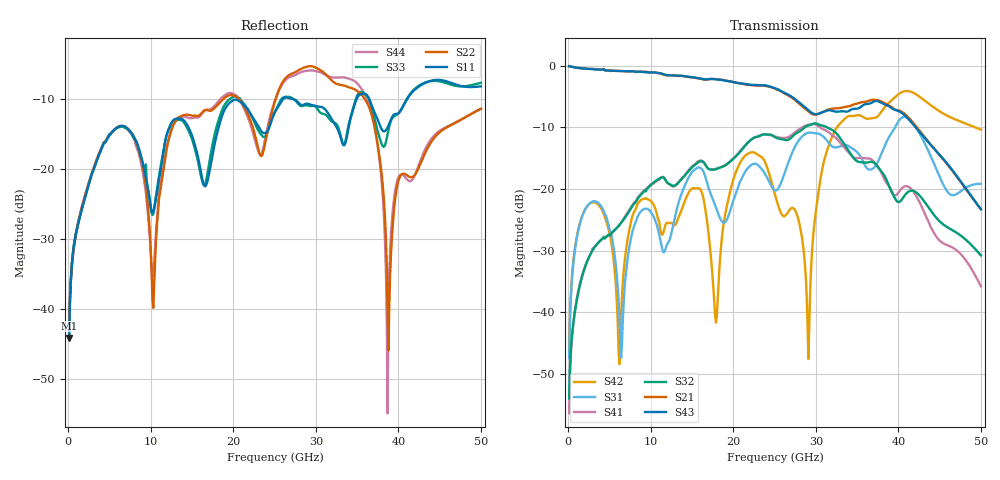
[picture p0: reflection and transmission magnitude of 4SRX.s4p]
! DAC39RF10ACK
! 256-pin FCBGA package
! Texas Instruments 8/20/2022
! Single-ended  S-parameters
! PORT#  PORT_NAME  NET_NAME
! PORT1:  xSRXN.DIEBUMP  xSRXN
! PORT2:  xSRXN.BGA  xSRXN
! PORT3:  xSRXP.DIEBUMP  xSRXP
! PORT4:  xSRXP.BGA  xSRXP
! Touchstone Ver. 1.0
! Number of ports is 4
# Hz	S	MA	R	50.000000
! SCATTERING PARAMETERS  :
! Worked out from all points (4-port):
!   500 points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, 100 MHz to 50 GHz, reference 50 ohm
!   strongest paths, dB at 100 MHz, 12.6 GHz, 25.1 GHz, 37.6 GHz, 50 GHz:
!     S43: 0.0, -1.6, -3.6, -5.8, -23.3
!     S21: 0.0, -1.6, -3.7, -5.6, -23.3
!     S32: -54.0, -19.4, -11.6, -16.5, -30.8
!     S41: -56.4, -19.6, -11.5, -16.5, -35.8
!     S31: -47.4, -26.6, -20.2, -15.3, -19.2
!     S42: -46.4, -25.6, -21.2, -8.1, -10.4
!   lowest |S11| = -44.1 dB at 100 MHz (marker M1), VSWR 1.01, Z = 50.5 + j0.403 ohm
!   |S11| at or under -10 dB: start of sweep to 26.11 GHz; 26.91 GHz to 34.98 GHz (8.066 GHz wide, 26.1 % of centre); 36.43 GHz to 41.11 GHz (4.673 GHz wide, 12.1 % of centre)
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1e8  0.006239 39.8  0.9862 -3.1  0.004188 84.3  0.001569 -63.0
     0.9949 -3.1  0.008032 25.0  0.001496 -101.9  0.004938 79.0
     0.004258 84.0  0.001997 -76.8  0.006477 40.5  0.9873 -3.4
     0.001513 -101.8  0.004769 80.1  0.9949 -3.1  0.009212 33.5
6.3e9  0.2009 -72.0  0.9073 -175.6  0.00599 -137.4  0.05199 91.8
       0.9096 -175.2  0.2015 -99.9  0.05223 92.4  0.006276 142.0
       0.005837 -141.3  0.05209 91.0  0.1988 -73.6  0.9062 -176.8
       0.05228 93.0  0.006112 143.6  0.9083 -176.2  0.1992 -100.1
1.28e10  0.2235 -99.9  0.8343 5.2  0.05491 155.0  0.1062 -94.1
         0.8358 5.1  0.2097 -69.6  0.1062 -96.3  0.05254 35.1
         0.05419 154.4  0.1063 -96.5  0.2172 -102.3  0.8355 2.8
         0.105 -94.2  0.05102 34.9  0.8357 2.9  0.2082 -72.6
1.91e10  0.2735 -39.8  0.7615 -169.7  0.05513 -176.0  0.158 98.3
         0.7615 -169.3  0.3245 -121.0  0.1571 96.1  0.06789 95.9
         0.05467 -175.7  0.1569 96.3  0.2939 -45.0  0.7572 -173.1
         0.1576 98.5  0.06685 94.5  0.7555 -173.0  0.3378 -121.8
3.54e10  0.338 -106.2  0.502 117.6  0.1827 -13.0  0.1787 -45.4
         0.5039 117.6  0.3429 151.5  0.1645 -54.9  0.3951 71.0
         0.1848 -14.4  0.1655 -55.7  0.3521 -108.6  0.4668 111.7
         0.1797 -45.2  0.3954 70.9  0.4622 112.3  0.3803 146.2
3.87e10  0.1968 -102.6  0.4846 12.9  0.2513 121.1  0.1087 -142.6
         0.4822 13.5  0.009954 103.1  0.1127 -154.1  0.4933 55.4
         0.2519 120.9  0.1125 -155.6  0.1766 -90.4  0.4765 4.8
         0.1092 -140.4  0.4907 55.3  0.4769 5.8  0.001811 -92.3
5e10  0.3859 -122.8  0.06336 113.0  0.1171 -32.8  0.03203 -17.6
      0.06872 124.6  0.267 -120.1  0.01344 -3.7  0.305 -33.2
      0.1103 -33.9  0.02892 -24.7  0.4091 -116.6  0.05506 100.1
      0.01625 -6.5  0.3037 -33.0  0.06854 116.0  0.2675 -121.2
